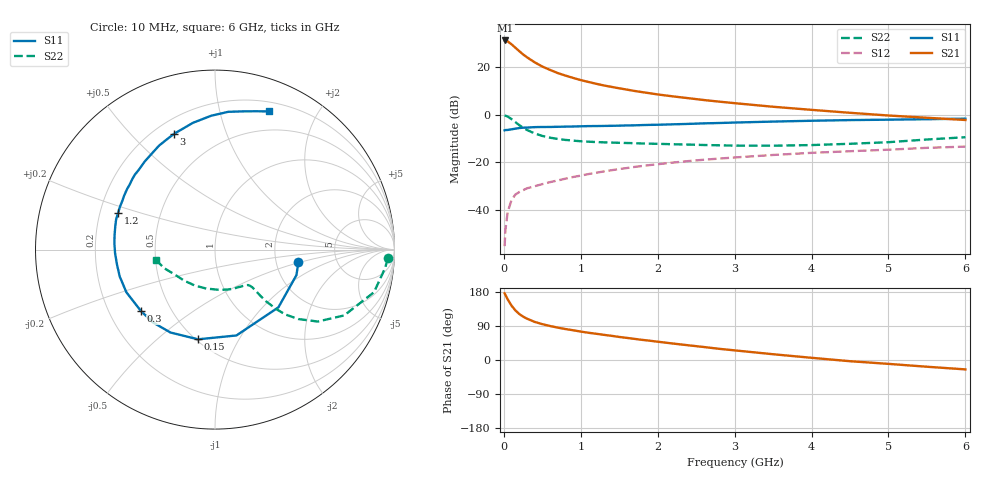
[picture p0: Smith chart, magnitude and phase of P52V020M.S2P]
! SIEMENS Small Signal Semiconductors
! BFP183
! Si NPN RF Bipolar Junction Transistor in SOT143
! VCE = 2 V  IC = 20 mA
! Common Emitter S-Parameters:  March  1996
# GHz  S  MA  R  50
!  f  S11  S21  S12  S22
! GHz  MAG  ANG  MAG  ANG  MAG  ANG  MAG  ANG
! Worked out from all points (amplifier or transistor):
!   36 points, 10 MHz to 6 GHz, reference 50 ohm
!   highest |S21| = 31.3 dB at 20 MHz (marker M1)
!   |S21| within 3 dB of that: start of sweep to 148.3 MHz
!   unconditionally stable (mu >= 1): 735.6 MHz to 5.582 GHz
!   at 250 MHz: K = 0.51, MSG = 28.6 dB, |S12| = -31.8 dB
!   at 1.4 GHz: K = 1.16, MAG = 15.1 dB, |S12| = -23.4 dB
!   at 6 GHz: K = 0.95, MSG = 5.6 dB, |S12| = -13.4 dB
!   S11 on the Smith chart (normalised r, x): 10 MHz: 2.67, -0.48; 150 MHz: 0.51, -0.69; 300 MHz: 0.34, -0.33; 1.2 GHz: 0.28, +0.17; 3 GHz: 0.28, +0.67; 6 GHz: 0.29, +1.43
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0.01  0.4699 -8.6  36.72 175.9  0.0017 82.8  0.9638 -2.9
0.02  0.4755 -17.4  36.73 172.1  0.0037 80.0  0.9538 -6.1
0.05  0.4778 -42.3  35.14 160.0  0.0089 77.8  0.9173 -15.0
0.1  0.4931 -76.0  30.48 143.5  0.016 62.1  0.8078 -27.0
0.15  0.5087 -100.7  25.85 130.9  0.0208 55.4  0.6986 -35.0
0.2  0.5245 -118.3  21.92 121.5  0.0234 52.0  0.6046 -39.8
0.25  0.5328 -130.3  18.68 114.5  0.0257 49.5  0.5328 -42.7
0.3  0.536 -140.2  16.26 109.2  0.0281 47.9  0.4776 -44.1
0.4  0.548 -154.3  12.74 100.6  0.0311 48.2  0.4042 -45.4
0.5  0.5517 -164.3  10.37 94.6  0.0345 49.0  0.3575 -45.5
0.6  0.5525 -171.6  8.812 89.7  0.038 49.5  0.3284 -45.3
0.7  0.5571 -178.0  7.555 85.5  0.0412 51.1  0.3088 -45.3
0.8  0.5614 176.7  6.691 81.7  0.0449 51.7  0.2948 -45.3
1.1  0.5761 163.0  4.904 71.9  0.0562 52.9  0.2702 -47.0
1.2  0.5772 159.2  4.49 69.3  0.0599 53.1  0.2659 -48.1
1.7  0.5979 142.6  3.167 55.7  0.0794 52.3  0.2511 -55.4
2.2  0.6279 128.6  2.434 43.4  0.0982 49.0  0.2389 -65.7
3  0.6845 109.4  1.752 25.4  0.1257 42.1  0.2233 -87.1
3.5  0.7172 99.8  1.472 15.2  0.1419 37.9  0.2224 -102.5
4.5  0.7712 84.5  1.098 -3.2  0.1703 28.7  0.2442 -135.1
5.5  0.8047 73.3  0.863 -17.8  0.2007 20.9  0.3005 -159.7
6  0.8267 68.6  0.775 -24.8  0.2129 16.1  0.336 -170.4
